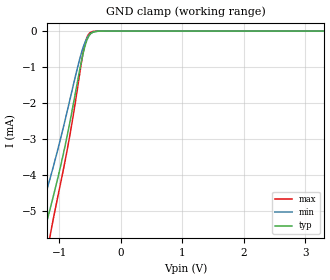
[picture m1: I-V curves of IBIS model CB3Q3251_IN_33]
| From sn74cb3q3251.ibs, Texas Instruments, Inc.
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[Model]   CB3Q3251_IN_33
Model_type  Input
Vinl=0.8
Vinh=2.0
| variable   typ   min   max
C_comp   2.60pF   2.32pF   2.77pF
[Temperature Range]   40   100   -40
| Ambient temperature   25   85   -40
[Voltage range]   3.3   3   3.6
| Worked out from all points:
|   GND clamp passes 1 mA (typ) near -0.66 V on its own axis
[GND Clamp]
| CB3Q3251_IN_33
|   Voltage   I(typ)   I(min)   I(max)
-5.5V     -49.44mA   -39.07mA   -64.15mA
-1.395V   -6.705mA   -5.604mA   -8.313mA
-1.245V   -5.549mA   -4.642mA   -6.598mA
-1.14V    -4.845mA   -4.006mA   -5.56mA
-985mV    -3.768mA   -3mA       -4.242mA
-840mV    -2.605mA   -1.972mA   -2.973mA
-705mV    -1.38mA    -1.001mA   -1.566mA
-605mV    -546.7uA   -401.6uA   -503.5uA
-555mV    -258uA     -201.9uA   -182.2uA
-505mV    -95.98uA   -84.4uA    -47.93uA
-380mV    -3.986uA   -5.274uA   -629.8nA
3.3V      73.51pA    242pA      26.64pA
